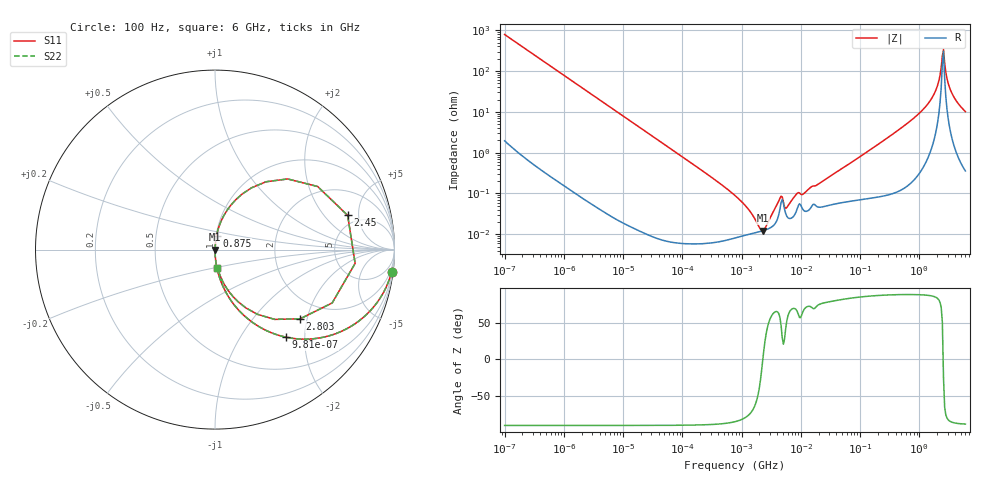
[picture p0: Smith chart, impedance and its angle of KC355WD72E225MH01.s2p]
!Murata Part Number: KC355WD72E225MH01
!These Parameters are Measured in Series Mode Connection
!Data Generated on Jun 19, 2026
!  o--ll--o
!Port1  Port2
!  o------o
!Operation Temp=25[degC], DC Bias Voltage=0[V]
!Freq. Start=100[Hz] Stop=6[GHz] 401[Steps]
# Hz S RI R 50
!Freq.(Hz) S11(Real) S11(Imag) S21(Real) S21(Imag) S12(Real) S12(Imag) S22(Real) S22(Imag)
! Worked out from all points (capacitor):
!   401 points, 100 Hz to 6 GHz, reference 50 ohm
!   read as one part in series: C = 2.02 uF near 109 Hz
!   lowest |Z| = 12.2 mohm at 2.269 MHz (marker M1)
!   series resonance near 2.284 MHz, so ESL is about 2.4 nH
!   S11 on the Smith chart (normalised r, x): 100 Hz: 1, -16; 981 Hz: 1.00, -1.61; 875 MHz: 1.00, +0.16; 2.45 GHz: 4.00, +3.65; 2.803 GHz: 1.47, -1.82; 6 GHz: 1.01, -0.20
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100  0.9839 -0.1248  0.0161 0.1248  0.0161 0.1248  0.9839 -0.1248
335  0.8469 -0.3591  0.1531 0.3591  0.1531 0.3591  0.8469 -0.3591
981  0.3938 -0.4876  0.6062 0.4876  0.6062 0.4876  0.3938 -0.4876
2008  0.1348 -0.3405  0.8652 0.3405  0.8652 0.3405  0.1348 -0.3405
7036  0.0128 -0.1111  0.9872 0.1111  0.9872 0.1111  0.0128 -0.1111
40335  0.000463 -0.0197  0.9995 0.0197  0.9995 0.0197  0.000463 -0.0197
774597  8.2e-05 -0.000888  0.9999 0.000888  0.9999 0.000888  8.2e-05 -0.000888
1267578  9.85e-05 -0.000421  0.9999 0.000421  0.9999 0.000421  9.85e-05 -0.000421
2268635  0.000122 -4.7e-06  0.9999 4.7e-06  0.9999 4.7e-06  0.000122 -4.7e-06
4440638  0.000414 0.00064  0.9996 -0.00064  0.9996 -0.00064  0.000414 0.00064
5809218  0.000276 0.000362  0.9997 -0.000362  0.9997 -0.000362  0.000276 0.000362
8692127  0.000421 0.000918  0.9996 -0.000918  0.9996 -0.000918  0.000421 0.000918
1.555665e7  0.000508 0.00141  0.9995 -0.00141  0.9995 -0.00141  0.000508 0.00141
3.124326e8  0.00155 0.0248  0.9984 -0.0248  0.9984 -0.0248  0.00155 0.0248
8.749838e8  0.00836 0.0769  0.9916 -0.0769  0.9916 -0.0769  0.00836 0.0769
1.791126e9  0.0893 0.2487  0.9107 -0.2487  0.9107 -0.2487  0.0893 0.2487
2.142435e9  0.2839 0.3779  0.7161 -0.3779  0.7161 -0.3779  0.2839 0.3779
2.450438e9  0.7391 0.1907  0.2609 -0.1907  0.2609 -0.1907  0.7391 0.1907
2.802721e9  0.4746 -0.3855  0.5254 0.3855  0.5254 0.3855  0.4746 -0.3855
3.065283e9  0.2354 -0.3602  0.7646 0.3602  0.7646 0.3602  0.2354 -0.3602
3.505958e9  0.0994 -0.2607  0.9006 0.2607  0.9006 0.2607  0.0994 -0.2607
6e9  0.0136 -0.0998  0.9864 0.0998  0.9864 0.0998  0.0136 -0.0998
